(* Logix 5000 AddOnInstructionDefinition export EH_iTherm_TM311_IOL; software revision 38.00 *)

TYPE EH_CommAOI_Data :
STRUCT
   Device_Comm_Error : BOOL;
   CommSuccess : BOOL;
   CommFailed : BOOL;
   CommTimeOut : BOOL;
   StateDone : BOOL;
   NewState : BOOL;
   OldState : SINT;
   PortSize : SINT;
   DevicePort : SINT;
   MaxState : SINT;
   State : SINT;
   VendorID : INT;
   DeviceID : DINT;
   CyclicData : INT[16];
   AcyclicData : DINT[8];
   ReplayIndex : INT;
   AOI_Diagnostic : DINT;
   ConnectionStatus : DINT;
   OutputData : INT[16];
END_STRUCT
END_TYPE

ADD_ON_INSTRUCTION EH_iTherm_TM311_IOL   (* revision 1.0, vendor Endress+Hauser *)
// iTherm TM311 Rev 1 IO-Link
VAR_IN_OUT
   DataToSend : INT[10]; {required}
   CommAOIBusy : DINT; {required}
   ActiveComPort : DINT; {required}
   DeviceAOISendRequest : DINT; {required}
   CommError : INT; {required}
   DeviceData : EH_CommAOI_Data; {required}
END_VAR
VAR_INPUT
   iExecuteRisingEdge : BOOL; {visible}
   iSetSimulation : BOOL; {visible}
   iSetSimulationTemperature : REAL; {visible}
   iSetUnit : DINT; {visible}   // 32 = °C // 33 = °F // 35 = K
END_VAR
VAR_OUTPUT
   qVendor_ID : DINT; {access Read Only, visible}
   qDevice_ID : DINT; {access Read Only, visible}
   qTemperature : REAL; {visible}
   qNegativOutOfRange : BOOL; {access Read Only, visible}
   qPositvOutOfRange : BOOL; {access Read Only, visible}
   qNoMeasurementData : BOOL; {access Read Only, visible}
   qSensorStatus : SINT; {visible}
   qS_Out_1 : BOOL; {access Read Only, visible}
   qSimulation : BOOL; {access Read Only, visible}
   qUnit : DINT; {access Read Only, visible}
   qAOI_Diagnostic : DINT; {access Read Only, visible}
END_VAR
VAR_IN_OUT
   qActual_Diagnostics_String : STRING; {required}
END_VAR
VAR_OUTPUT
   qActual_Diagnostics_Code : DINT; {access Read Only, visible}
END_VAR
VAR_IN_OUT
   qLast_Diagnostics_String : STRING; {required}
END_VAR
VAR_OUTPUT
   qLast_Diagnostics_Code : DINT; {access Read Only, visible}
   qCommunicationBusy : DINT; {access Read Only, visible}
   qCommError : INT; {access None, visible}
   qDeviceConnectionError : BOOL; {access Read Only, visible}
END_VAR
VAR
   Calc_DID : DINT; {access None}
   Calc_VID : DINT; {access None}
   Calc_Data : DINT; {access None}
   Temperature_INT : INT; {access None}
   CMD_Index : INT; {access None}
   Calc_Temperature : DINT; {access None}
   Calc_CondenStatus : DINT; {access None}
   CMD_Subindex : INT; {access None}
   CMD_ByteLength : INT; {access None}
   Trigger : BOOL; {access None}
   CMD_Rd : BOOL; {access None}
   CMD_Wr : BOOL; {access None}
   Calc_Out : DINT; {access None}
   UnitSelection : REAL; {access None}
   InputByteLength : DINT;
   SimulationDINT : DINT; {access None}
   StateMin : INT; {access None}
   qDevice_ID_select : INT; {access None}
   UseDeviceUnit : BOOL; {access None}
   AOI_Prio : BOOL; {access None}
   ActiveAOI : BOOL; {access None}
   firstTimeDone : BOOL; {access None}
   Scale_SINT : DINT; {access None}
   DeviceID1 : DINT; {access None}
   DeviceID2 : DINT; {access None}
   TRUE : BOOL := 1; {access None}
   FALSE : BOOL; {access None}
   WrongDeviceID : BOOL; {access None}
END_VAR

ROUTINE Logic   (* structured text *)
// PMP23 Communication via AL1323
   // ©Copyright (2024) All Rights Reserved
   // =======================================================================
   // Name:                EH_iTherm_TM311_IOL
   // Version:             1.0
   // Datum:               11.2025
   // Library:             01.01.00
   // Engineering:         Studio5000 V38.00.00
   // Author:              EH
   // =======================================================================
   
   
   qAOI_Diagnostic := DeviceData.AOI_Diagnostic;
   qCommunicationBusy := CommAOIBusy;
   DeviceID1 := 196864; // TM311
   DeviceID2 := 8585472; // OTM311
   StateMin := 0;
   DeviceData.MaxState := 8;
   
   if DeviceData.DeviceID = DeviceID1 or DeviceData.DeviceID = DeviceID2 then
   
   	WrongDeviceID := FALSE;
   else
   
   	WrongDeviceID := TRUE;
   
   end_if;
   
   if DeviceData.DevicePort = 0 or WrongDeviceID or DeviceData.ConnectionStatus <> 1 then
   
   	qVendor_ID	:= 0;
   	qDevice_ID	:= 0;
   	qTemperature:= 0;
   	qS_Out_1	:= 0;
   	qSimulation	:= 0;
   	qUnit	:= 0;
   	qSensorStatus	:= 0;
   	qActual_Diagnostics_Code	:= 0;
   	qLast_Diagnostics_Code	:= 0;
   	qLast_Diagnostics_String	:= '';
   
   	if DeviceData.DevicePort = 0 then
   
   		qActual_Diagnostics_String	:= 'Device Port is Zero';
   		DeviceData.AOI_Diagnostic.1 := TRUE;
   
   	elsif DeviceData.ConnectionStatus <> 1 then
   
   		qActual_Diagnostics_String	:= 'No Device connected';
   		qDeviceConnectionError := TRUE;
   
   	elsif WrongDeviceID then
   
   		qActual_Diagnostics_String	:= 'Wrong DeviceID';
   		DeviceData.AOI_Diagnostic.2 := TRUE;
   		qVendor_ID := DeviceData.VendorID;
   		qDevice_ID := DeviceData.DeviceID;
   
   	end_if;
   
   else
   
   	if qActual_Diagnostics_Code = 0 then
   
   		qActual_Diagnostics_String	:= '--------';
   
   	end_if;
   
   	if qLast_Diagnostics_Code = 0 then
   
   		qLast_Diagnostics_String	:= '--------';
   
   	end_if;
   
   	DeviceData.AOI_Diagnostic.1 := FALSE;
   	qDeviceConnectionError := FALSE;
   	DeviceData.AOI_Diagnostic.2  := FALSE;
   
   end_if;
   
   
   if not DeviceData.AOI_Diagnostic.0
   	and not qDeviceConnectionError
   	and not DeviceData.AOI_Diagnostic.2
   	and DeviceData.DevicePort > 0 or ActiveAOI and qDeviceConnectionError then
   
   	//*********************************
   	//Vendor ID
   	//*********************************
   
   	qVendor_ID := DeviceData.VendorID;
   
   	//*********************************
   	//Device ID
   	//*********************************
   
   	qDevice_ID := DeviceData.DeviceID;
   
   	//*********************************
   	//Process Data Temperature
   	//*********************************
   	if DeviceData.DeviceID = DeviceID1 then
   
   		qDevice_ID_select := 1;
   
   	elsif DeviceData.DeviceID = DeviceID2 then
   
   		qDevice_ID_select := 2;
   
   	else
   
   		qDevice_ID_select := 0;
   
   	end_if;
   
   	Calc_Temperature := 0+((DeviceData.DevicePort-1)*InputByteLength);
   
   	case qDevice_ID_select of				// Selection of the Process Data according to the Device ID
   
   		//*********************************
   		1: // TM311
   		//*********************************
   
   		Temperature_INT := DeviceData.CyclicData[Calc_Temperature];
   
   		Scale_SINT.0 := DeviceData.CyclicData[Calc_Temperature+1].8;
   		Scale_SINT.1 := DeviceData.CyclicData[Calc_Temperature+1].9;
   		Scale_SINT.2 := DeviceData.CyclicData[Calc_Temperature+1].10;
   		Scale_SINT.3 := DeviceData.CyclicData[Calc_Temperature+1].11;
   		Scale_SINT.4 := DeviceData.CyclicData[Calc_Temperature+1].12;
   		Scale_SINT.5 := DeviceData.CyclicData[Calc_Temperature+1].13;
   		Scale_SINT.6 := DeviceData.CyclicData[Calc_Temperature+1].14;
   		Scale_SINT.7 := DeviceData.CyclicData[Calc_Temperature+1].15;
   
   		UnitSelection := Scale_SINT;
   
   		//*********************************
   		2: // OTM311
   		//*********************************
   
   		Temperature_INT := DeviceData.CyclicData[Calc_Temperature];
   
   		Scale_SINT.0 := DeviceData.CyclicData[Calc_Temperature+1].8;
   		Scale_SINT.1 := DeviceData.CyclicData[Calc_Temperature+1].9;
   		Scale_SINT.2 := DeviceData.CyclicData[Calc_Temperature+1].10;
   		Scale_SINT.3 := DeviceData.CyclicData[Calc_Temperature+1].11;
   		Scale_SINT.4 := DeviceData.CyclicData[Calc_Temperature+1].12;
   		Scale_SINT.5 := DeviceData.CyclicData[Calc_Temperature+1].13;
   		Scale_SINT.6 := DeviceData.CyclicData[Calc_Temperature+1].14;
   		Scale_SINT.7 := DeviceData.CyclicData[Calc_Temperature+1].15;
   
   		UnitSelection := Scale_SINT;
   
   	end_case;
   
   		if Temperature_INT = -32760 then
   
   			qNegativOutOfRange := 1;
   			qPositvOutOfRange :=0;
   			qNoMeasurementData := 0;
   
   		elsif Temperature_INT = 32760 then
   
   			qNegativOutOfRange := 0;
   			qPositvOutOfRange :=1;
   			qNoMeasurementData := 0;
   
   		elsif Temperature_INT = 32764 then
   
   			qNegativOutOfRange := 0;
   			qPositvOutOfRange :=0;
   			qNoMeasurementData := 1;
   
   		else
   
   			qNegativOutOfRange := 0;
   			qPositvOutOfRange :=0;
   			qNoMeasurementData := 0;
   
   		end_if;
   
   		if UnitSelection = 255 then
   
   			qTemperature := Temperature_INT;
   			qTemperature := qTemperature / 10;  // scale = 10 ^(scale) -->  10^(-1) = 0.1 --> Value*0.1 == Value/10
   			DeviceData.AOI_Diagnostic.2 := 0;
   		else
   
   			DeviceData.AOI_Diagnostic.2 := 1;				// Manual states that the Scale is only -1 so error should not accure
   
   		end_if;
   
   
   
   	//*********************************
   	// Process Parameter State IO1
   	//*********************************
   
   		if qDevice_ID = DeviceID1 then				// selection of the Switch State for the different Devcie ID
   
   			qS_Out_1 := DeviceData.CyclicData[Calc_Temperature+1].0;
   
   		elsif qDevice_ID = DeviceID2 then
   
   			qS_Out_1 := DeviceData.CyclicData[Calc_Temperature+1].0;
   
   		end_if;
   
   	//*********************************
   	// Sensor status
   	//*********************************
   
   		qSensorStatus.0 := DeviceData.CyclicData[Calc_Temperature+1].1;
   		qSensorStatus.1 := DeviceData.CyclicData[Calc_Temperature+1].2;
   		qSensorStatus.2 := DeviceData.CyclicData[Calc_Temperature+1].3;
   		qSensorStatus.3 := DeviceData.CyclicData[Calc_Temperature+1].4;
   
   	//*********************************
   	// Checking for CommBlockBusy
   	//*********************************
   
   	if iExecuteRisingEdge and DeviceData.State = 0 then
   
   		DeviceAOISendRequest.[DeviceData.DevicePort] := 1;
   
   	end_if;
   
   	if ActiveComPort = DeviceData.DevicePort then
   
   		AOI_Prio :=1;
   	else
   
   		AOI_Prio := 0;
   	end_if;
   
   
   	if CommAOIBusy = 1 and iExecuteRisingEdge and DeviceData.State = 0 and AOI_Prio then
   
   		ActiveAOI := 1;
   
   	end_if;
   
   	qCommunicationBusy := CommAOIBusy;
   	qAOI_Diagnostic := DeviceData.AOI_Diagnostic;
   
   	if  ActiveAOI and qDeviceConnectionError then
   
   		DeviceData.State := DeviceData.MaxState;
   
   	end_if;
   
   
   	//*********************************
   	// State machine
   	//*********************************
   
   	if ActiveAOI or DeviceData.State = DeviceData.MaxState then
   
   		case DeviceData.State of
   
   			//*********************************
   			0: // Idle
   			//*********************************
   
   			// Initializing this state is the starting State / Idle State for the State Machinge
   				Trigger := 0;
   				CMD_Index := 0;
   				CMD_Subindex := 0;
   				CMD_Wr := 0;
   				CMD_Rd := 0;
   				CMD_ByteLength := 0;
   
   
   				if DeviceData.DevicePort = ActiveComPort then // check if Device is Active to reset success
   					DeviceData.CommSuccess := 0;
   					DeviceData.CommTimeOut := 0;
   					DeviceData.NewState := 1;
   					DeviceData.StateDone := 0;
   				end_if;
   
   			    // Wait for trigger
   			    if iExecuteRisingEdge and ActiveComPort = DeviceData.DevicePort then
   
   					DeviceData.AOI_Diagnostic := 0;
   					DeviceData.State := DeviceData.State + 1;
   
   			    end_if;
   
   			//*********************************
   			1: // Set Unit
   			//*********************************
   
   				CMD_Index := 5121;
   				CMD_Subindex := 0;
   				CMD_Wr := 1;									// Only Read or Write can be active = 1
   				CMD_Rd := 0;
   				CMD_ByteLength := 1;
   				DataToSend[6]:= 0;
   				DataToSend[7]:= 0;
   
   			if iSetUnit >= 32 AND iSetUnit <= 35 then			// Check if the value from outside is usable if not error set an go to next Step
   
   				DataToSend[6].0 := iSetUnit.0;			// 32 = °C ; 33 = °F ; 35 = K
   				DataToSend[6].1 := iSetUnit.1;
   				DataToSend[6].2 := iSetUnit.2;
   				DataToSend[6].3 := iSetUnit.3;
   				DataToSend[6].4 := iSetUnit.4;
   				DataToSend[6].5 := iSetUnit.5;
   				DataToSend[6].6 := iSetUnit.6;
   				DataToSend[6].7 := iSetUnit.7;
   
   				Trigger := 1;
   
   				if DeviceData.NewState then
   
   					DeviceData.StateDone := 1;
   
   				end_if;
   
   				if  DeviceData.CommSuccess and DeviceData.ReplayIndex = CMD_Index then
   
   					Trigger := 0;
   					DeviceData.OldState := DeviceData.State;
   			        DeviceData.State := DeviceData.State + 1;
   					DeviceData.CommSuccess := 0;
   					DeviceData.AcyclicData[0] := 0;
   					DeviceData.NewState := 1;
   
   				 elsif DeviceData.CommTimeOut then
   
   					DeviceData.AOI_Diagnostic.[DeviceData.State+7] := 1;
   					DeviceData.OldState := DeviceData.State;
   			        DeviceData.State := DeviceData.State + 1;
   					DeviceData.CommTimeOut := 0;
   					DeviceData.AcyclicData[0] := 0;
   					DeviceData.NewState := 1;
   
   			    end_if;
   
   				else
   
   					DeviceData.AOI_Diagnostic.[DeviceData.State+7] := 1;
   					DeviceData.OldState := DeviceData.State;
   			        DeviceData.State := DeviceData.State + 1;
   					DeviceData.CommTimeOut := 0;
   					DeviceData.AcyclicData[0] := 0;
   					DeviceData.NewState := 1;
   
   				end_if;
   
   			//*********************************
   			2: // Set Simulation Value Temperature
   			//*********************************
   
   				CMD_Index := 3104;
   				CMD_Subindex := 0;
   				CMD_Wr := 1;
   				CMD_Rd := 0;
   				CMD_ByteLength := 4;
   
   				COP(iSetSimulationTemperature,SimulationDINT,1); // Copy the Bits of the REAL in a DINT not the Value
   
   				DataToSend[6].0 :=  SimulationDINT.24;
   				DataToSend[6].1 :=  SimulationDINT.25;
   				DataToSend[6].2 :=  SimulationDINT.26;
   				DataToSend[6].3 :=  SimulationDINT.27;
   				DataToSend[6].4 :=  SimulationDINT.28;
   				DataToSend[6].5 :=  SimulationDINT.29;
   				DataToSend[6].6 :=  SimulationDINT.30;
   				DataToSend[6].7 :=  SimulationDINT.31;
   				DataToSend[6].8 :=  SimulationDINT.16;
   				DataToSend[6].9 :=  SimulationDINT.17;
   				DataToSend[6].10 := SimulationDINT.18;
   				DataToSend[6].11 := SimulationDINT.19;
   				DataToSend[6].12 := SimulationDINT.20;
   				DataToSend[6].13 := SimulationDINT.21;
   				DataToSend[6].14 := SimulationDINT.22;
   				DataToSend[6].15 := SimulationDINT.23;
   				DataToSend[7].0  := SimulationDINT.8;
   				DataToSend[7].1  := SimulationDINT.9;
   				DataToSend[7].2  := SimulationDINT.10;
   				DataToSend[7].3  := SimulationDINT.11;
   				DataToSend[7].4  := SimulationDINT.12;
   				DataToSend[7].5  := SimulationDINT.13;
   				DataToSend[7].6  := SimulationDINT.14;
   				DataToSend[7].7  := SimulationDINT.15;
   				DataToSend[7].8  := SimulationDINT.0;
   				DataToSend[7].9  := SimulationDINT.1;
   				DataToSend[7].10 := SimulationDINT.2;
   				DataToSend[7].11 := SimulationDINT.3;
   				DataToSend[7].12 := SimulationDINT.4;
   				DataToSend[7].13 := SimulationDINT.5;
   				DataToSend[7].14 := SimulationDINT.6;
   				DataToSend[7].15 := SimulationDINT.7;
   
   				Trigger := 1;
   
   				if DeviceData.NewState then
   
   					DeviceData.StateDone := 1;
   
   				end_if;
   
   				if  DeviceData.CommSuccess and DeviceData.ReplayIndex = CMD_Index then
   
   						Trigger := 0;
   						DeviceData.OldState := DeviceData.State;
   				        DeviceData.State := DeviceData.State + 1;
   						DeviceData.CommSuccess := 0;
   						DeviceData.AcyclicData[0] := 0;
   						DeviceData.NewState := 1;
   
   				 elsif DeviceData.CommTimeOut then
   
   						DeviceData.AOI_Diagnostic.[DeviceData.State+7] := 1;
   						DeviceData.OldState := DeviceData.State;
   				        DeviceData.State := DeviceData.State + 1;
   						DeviceData.CommTimeOut := 0;
   						DeviceData.AcyclicData[0] := 0;
   						DeviceData.NewState := 1;
   
   				   end_if;
   
   			//*********************************
   			3: // Set Simulation
   			//*********************************
   
   				CMD_Index := 3109;
   				CMD_Subindex := 0;
   				CMD_Wr := 1;
   				CMD_Rd := 0;
   				CMD_ByteLength := 1;
   				DataToSend[6]:= 0;
   				DataToSend[7]:= 0;
   
   				DataToSend[6].0 := iSetSimulation;
   				Trigger := 1;
   
   				if DeviceData.NewState then
   
   					DeviceData.StateDone := 1;
   
   				end_if;
   
   				if  DeviceData.CommSuccess and DeviceData.ReplayIndex = CMD_Index then
   
   					Trigger := 0;
   					DeviceData.OldState := DeviceData.State;
   			        DeviceData.State := DeviceData.State + 1;
   					DeviceData.CommSuccess := 0;
   					DeviceData.AcyclicData[0] := 0;
   					DeviceData.NewState := 1;
   
   				 elsif DeviceData.CommTimeOut then
   
   					DeviceData.AOI_Diagnostic.[DeviceData.State+7] := 1;
   					DeviceData.OldState := DeviceData.State;
   			        DeviceData.State := DeviceData.State + 1;
   					DeviceData.CommTimeOut := 0;
   					DeviceData.AcyclicData[0] := 0;
   					DeviceData.NewState := 1;
   
   			    end_if;
   
   			//*********************************
   			4: // Read Unit Set from Device
   			//*********************************
   
   				CMD_Index := 5121;
   				CMD_Subindex := 0;
   				CMD_Wr := 0;
   				CMD_Rd := 1;
   				CMD_ByteLength := 1;
   				DataToSend[6]:= 0;
   				DataToSend[7]:= 0;
   				Trigger := 1;
   
   				if DeviceData.NewState then
   
   					DeviceData.StateDone := 1;
   
   				end_if;
   
   				if  DeviceData.CommSuccess and DeviceData.ReplayIndex = CMD_Index then
   
   					qUnit.0 := DeviceData.AcyclicData[0].0;
   					qUnit.1 := DeviceData.AcyclicData[0].1;
   					qUnit.2 := DeviceData.AcyclicData[0].2;
   					qUnit.3 := DeviceData.AcyclicData[0].3;
   					qUnit.4 := DeviceData.AcyclicData[0].4;
   					qUnit.5 := DeviceData.AcyclicData[0].5;
   					qUnit.6 := DeviceData.AcyclicData[0].6;
   					qUnit.7 := DeviceData.AcyclicData[0].7;
   
   					UseDeviceUnit := 1;
   					Trigger := 0;
   					DeviceData.OldState := DeviceData.State;
   			        DeviceData.State := DeviceData.State + 1;
   					DeviceData.CommSuccess := 0;
   					DeviceData.AcyclicData[0] := 0;
   					DeviceData.NewState := 1;
   
   				 elsif DeviceData.CommTimeOut then
   
   					DeviceData.AOI_Diagnostic.[DeviceData.State+7] := 1;
   					DeviceData.OldState := DeviceData.State;
   			        DeviceData.State := DeviceData.State + 1;
   					DeviceData.CommTimeOut := 0;
   					DeviceData.AcyclicData[0] := 0;
   					DeviceData.NewState := 1;
   
   			    end_if;
   
   			//*********************************
   			5: // Read Simulation Active
   			//*********************************
   
   				CMD_Index := 3109;
   				CMD_Subindex := 0;
   				CMD_Wr := 0;
   				CMD_Rd := 1;
   				CMD_ByteLength := 1;
   				DataToSend[6]:= 0;
   				DataToSend[7]:= 0;
   				Trigger := 1;
   
   				if DeviceData.NewState then
   					DeviceData.StateDone := 1;
   				end_if;
   
   				if  DeviceData.CommSuccess and DeviceData.ReplayIndex = CMD_Index then
   
   					qSimulation := DeviceData.AcyclicData[0].0;
   
   					Trigger := 0;
   					DeviceData.OldState := DeviceData.State;
   			        DeviceData.State := DeviceData.State + 1;
   					DeviceData.CommSuccess := 0;
   					DeviceData.AcyclicData[0] := 0;
   					DeviceData.NewState := 1;
   
   				elsif DeviceData.CommTimeOut then
   
   					DeviceData.AOI_Diagnostic.[DeviceData.State+7] := 1;
   					Trigger := 0;
   					DeviceData.OldState := DeviceData.State;
   			        DeviceData.State := DeviceData.State + 1;
   					DeviceData.CommTimeOut := 0;
   					DeviceData.AcyclicData[0] := 0;
   					DeviceData.NewState := 1;
   
   			    end_if;
   
   			//*********************************
   			6: // Actual Diagnostic
   			//*********************************
   
   				CMD_Index := 6184;
   				CMD_Subindex := 0;
   				CMD_Wr := 0;
   				CMD_Rd := 1;
   				CMD_ByteLength := 2;
   				Trigger := 1;
   
   				if DeviceData.NewState then
   
   				DeviceData.StateDone := 1;
   
   				end_if;
   
   				if  DeviceData.CommSuccess and DeviceData.ReplayIndex = CMD_Index then
   
   					qActual_Diagnostics_Code	:= DeviceData.AcyclicData[0];
   
   					case qActual_Diagnostics_Code of
   
   						16#0000_0000:
   							qActual_Diagnostics_String := 'System ok';
   						16#0000_0001:
   							qActual_Diagnostics_String := 'no communication';
   						16#0000_4001:
   							qActual_Diagnostics_String := 'F001 - Device failure';
   						16#0000_4004:
   							qActual_Diagnostics_String := 'F004 - Sensor defective';
   						16#0000_102F:
   							qActual_Diagnostics_String := 'S047 - Sensor limit reached';
   						16#0000_2191:
   							qActual_Diagnostics_String := 'C401 - Factory Reset active';
   						16#0000_2192:
   							qActual_Diagnostics_String := 'C402 + Initialization active';
   						16#0000_21E5:
   							qActual_Diagnostics_String := 'C485 - Process varable sim. active';
   						16#0000_21E8:
   							qActual_Diagnostics_String := 'C491 + Current output sim. active';
   						16#0000_21EE:
   							qActual_Diagnostics_String := 'C494 - Switch output sim. active';
   						16#0000_4219:
   							qActual_Diagnostics_String := 'F537 - Configuration invalid';
   						16#0000_1321:
   							qActual_Diagnostics_String := 'S801 - Supply voltage too low';
   						16#0000_1324:
   							qActual_Diagnostics_String := 'S804 - Overload at switch output';
   						16#0000_1339:
   							qActual_Diagnostics_String := 'S825 - Operating temperature';
   						16#0000_134C:
   							qActual_Diagnostics_String := 'S844 - Process value out of spec.';
   						else
   							qActual_Diagnostics_String := 'Error Code unknown';
   
   			 		end_case;
   
   					Trigger := 0;
   					DeviceData.OldState := DeviceData.State;
   			        DeviceData.State := DeviceData.State + 1;
   					DeviceData.CommSuccess := 0;
   					DeviceData.AcyclicData[0] := 0;
   					DeviceData.NewState := 1;
   
   				elsif DeviceData.CommTimeOut then
   
   					DeviceData.AOI_Diagnostic.[DeviceData.State+7] := 1;
   					Trigger := 0;
   					DeviceData.OldState := DeviceData.State;
   			        DeviceData.State := DeviceData.State + 1;
   					DeviceData.CommTimeOut := 0;
   					DeviceData.AcyclicData[0] := 0;
   					DeviceData.NewState := 1;
   
   			    end_if;
   
   			//*********************************
   			7: // Last Diagnostic
   			//*********************************
   
   				CMD_Index := 6214;
   				CMD_Subindex := 0;
   				CMD_Wr := 0;
   				CMD_Rd := 1;
   				CMD_ByteLength := 2;
   				Trigger := 1;
   
   				if DeviceData.NewState then
   
   					DeviceData.StateDone := 1;
   
   				end_if;
   
   				if  DeviceData.CommSuccess and DeviceData.ReplayIndex = CMD_Index then
   
   					qLast_Diagnostics_Code	:= DeviceData.AcyclicData[0];
   
   					case qLast_Diagnostics_Code of
   
   						16#0000_0000:
   							qLast_Diagnostics_String := 'System ok';
   						16#0001_0000:
   							qLast_Diagnostics_String := 'no communication';
   						16#0000_4001:
   							qLast_Diagnostics_String := 'F001 - Device failure';
   						16#0000_4004:
   							qLast_Diagnostics_String := 'F004 - Sensor defective';
   						16#0000_102F:
   							qLast_Diagnostics_String := 'S047 - Sensor limit reached';
   						16#0000_2191:
   							qLast_Diagnostics_String := 'C401 - Factory Reset active';
   						16#0000_2192:
   							qLast_Diagnostics_String := 'C402 + Initialization active';
   						16#0000_21E5:
   							qLast_Diagnostics_String := 'C485 - Process varable sim. active';
   						16#0000_21E8:
   							qLast_Diagnostics_String := 'C491 + Current output sim. active';
   						16#0000_21EE:
   							qLast_Diagnostics_String := 'C494 - Switch output sim. active';
   						16#0000_4219:
   							qLast_Diagnostics_String := 'F537 - Configuration invalid';
   						16#0000_1321:
   							qLast_Diagnostics_String := 'S801 - Supply voltage too low';
   						16#0000_1324:
   							qLast_Diagnostics_String := 'S804 - Overload at switch output';
   						16#0000_1339:
   							qLast_Diagnostics_String := 'S825 - Operating temperature';
   						16#0000_134C:
   							qLast_Diagnostics_String := 'S844 - Process value out of spec.';
   						else
   							qLast_Diagnostics_String := 'Error Code unknown';
   
   			 		end_case;
   
   					Trigger := 0;
   					DeviceData.OldState := DeviceData.State;
   			        DeviceData.State := DeviceData.State + 1;
   					DeviceData.CommSuccess := 0;
   					DeviceData.AcyclicData[0] := 0;
   					DeviceData.NewState := 1;
   
   				elsif DeviceData.CommTimeOut then
   
   					DeviceData.AOI_Diagnostic.[DeviceData.State+7] := 1;
   					Trigger := 0;
   					DeviceData.OldState := DeviceData.State;
   			        DeviceData.State := DeviceData.State + 1;
   					DeviceData.CommTimeOut := 0;
   					DeviceData.AcyclicData[0] := 0;
   					DeviceData.NewState := 1;
   
   			    end_if;
   
   			//*********************************
   			8: // Tigger guard
   			//*********************************
   
   				if not firstTimeDone then
   
   					CommAOIBusy := 0;
   					firstTimeDone := 1;
   					DeviceAOISendRequest.[DeviceData.DevicePort] := 0;
   					ActiveComPort := 0;
   					ActiveAOI := 0;
   					DataToSend[0] := 0;
   					DataToSend[1] := 0;
   					DataToSend[2] := 0;
   					DataToSend[3] := 0;
   					DataToSend[4] := 0;
   					DataToSend[5] := 0;
   					DataToSend[6] := 0;
   					DataToSend[7] := 0;
   					DataToSend[8] := 0;
   					DataToSend[9] := 0;
   					DeviceData.StateDone := 0;
   
   				end_if;
   
   				if DeviceData.State = DeviceData.MaxState AND NOT iExecuteRisingEdge then
   
   					DeviceData.State := 0;
   					DeviceData.OldState := DeviceData.State;
   					firstTimeDone := 0;
   
   				end_if;
   
   			end_case;
   
   		end_if;
   
   	//*************************
   	// Write Commands to the Master and the Device
   	//*************************
   
   	if DeviceData.State > StateMin and DeviceData.State < DeviceData.MaxState then
   
   		DataToSend[2] :=  DeviceData.DevicePort;		// Port from @ the IFM Master
   		DataToSend[3] := CMD_Index;			// Command Index No.
   		DataToSend[4] := CMD_Subindex;		// Subindex No.
   		DataToSend[5].0 := CMD_Rd;			// If 1 the Command is Read only Read or Write can be 1
   		DataToSend[5].1 := CMD_Wr;			// If 1 the Command is Write
   		DataToSend[5].8 := CMD_ByteLength.0;  // Bits for Data Length
   		DataToSend[5].9 := CMD_ByteLength.1;
   		DataToSend[5].10 := CMD_ByteLength.2;
   		DataToSend[5].11 := CMD_ByteLength.3;
   		DataToSend[5].12 := CMD_ByteLength.4;
   		DataToSend[5].13 := CMD_ByteLength.5;
   		DataToSend[5].14 := CMD_ByteLength.6;
   		DataToSend[5].15 := CMD_ByteLength.7;
   
   		DataToSend[5].7 := Trigger;
   
   		qCommError	:= CommError;
   
   	end_if;
   
   end_if;
   
END_ROUTINE
END_ADD_ON_INSTRUCTION
